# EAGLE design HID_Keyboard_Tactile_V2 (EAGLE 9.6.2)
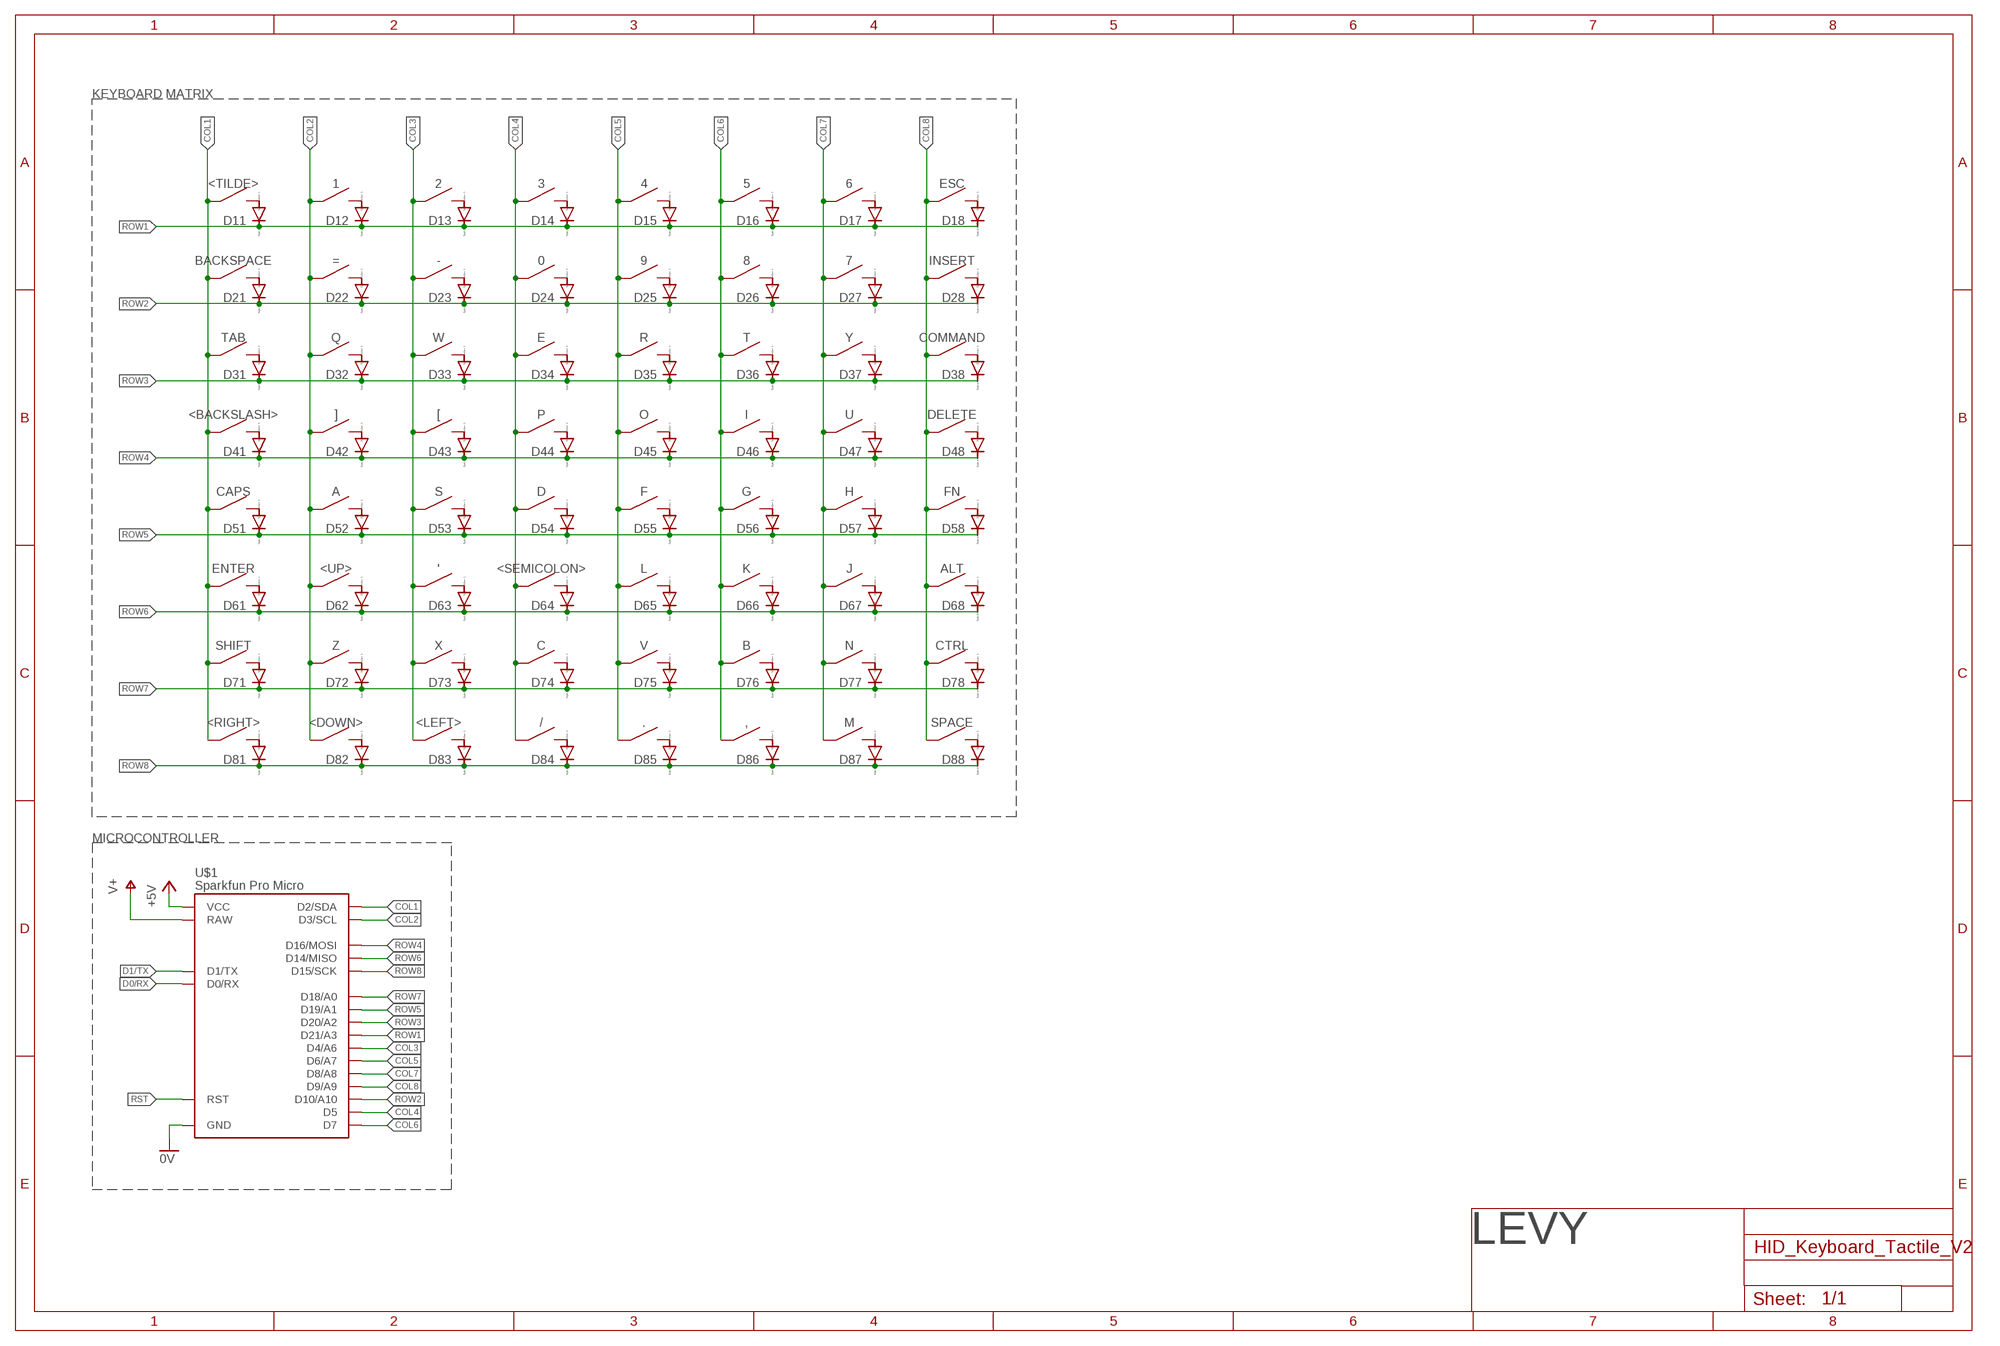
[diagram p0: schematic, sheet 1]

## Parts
0  KEYBOARD_KEYTACTILE_16MM  [KEYBOARD_KEY_TACTILE]
1  KEYBOARD_KEYTACTILE_16MM  [KEYBOARD_KEY_TACTILE]
2  KEYBOARD_KEYTACTILE_16MM  [KEYBOARD_KEY_TACTILE]
3  KEYBOARD_KEYTACTILE_16MM  [KEYBOARD_KEY_TACTILE]
4  KEYBOARD_KEYTACTILE_16MM  [KEYBOARD_KEY_TACTILE]
5  KEYBOARD_KEYTACTILE_16MM  [KEYBOARD_KEY_TACTILE]
6  KEYBOARD_KEYTACTILE_16MM  [KEYBOARD_KEY_TACTILE]
7  KEYBOARD_KEYTACTILE_16MM  [KEYBOARD_KEY_TACTILE]
8  KEYBOARD_KEYTACTILE_16MM  [KEYBOARD_KEY_TACTILE]
9  KEYBOARD_KEYTACTILE_16MM  [KEYBOARD_KEY_TACTILE]
'  KEYBOARD_KEYTACTILE_16MM  [KEYBOARD_KEY_TACTILE]
,  KEYBOARD_KEYTACTILE_16MM  [KEYBOARD_KEY_TACTILE]
-  KEYBOARD_KEYTACTILE_16MM  [KEYBOARD_KEY_TACTILE]
.  KEYBOARD_KEYTACTILE_16MM  [KEYBOARD_KEY_TACTILE]
/  KEYBOARD_KEYTACTILE_16MM  [KEYBOARD_KEY_TACTILE]
<BACKSLASH>  KEYBOARD_KEYTACTILE_16MM  [KEYBOARD_KEY_TACTILE]
<DOWN>  KEYBOARD_KEYTACTILE_16MM  [KEYBOARD_KEY_TACTILE]
<LEFT>  KEYBOARD_KEYTACTILE_16MM  [KEYBOARD_KEY_TACTILE]
<RIGHT>  KEYBOARD_KEYTACTILE_16MM  [KEYBOARD_KEY_TACTILE]
<SEMICOLON>  KEYBOARD_KEYTACTILE_16MM  [KEYBOARD_KEY_TACTILE]
<TILDE>  KEYBOARD_KEYTACTILE_16MM  [KEYBOARD_KEY_TACTILE]
<UP>  KEYBOARD_KEYTACTILE_16MM  [KEYBOARD_KEY_TACTILE]
=  KEYBOARD_KEYTACTILE_16MM  [KEYBOARD_KEY_TACTILE]
[  KEYBOARD_KEYTACTILE_16MM  [KEYBOARD_KEY_TACTILE]
]  KEYBOARD_KEYTACTILE_16MM  [KEYBOARD_KEY_TACTILE]
A  KEYBOARD_KEYTACTILE_16MM  [KEYBOARD_KEY_TACTILE]
ALT  KEYBOARD_KEYTACTILE_16MM  [KEYBOARD_KEY_TACTILE]
B  KEYBOARD_KEYTACTILE_16MM  [KEYBOARD_KEY_TACTILE]
BACKSPACE  KEYBOARD_KEYTACTILE_16MM  [KEYBOARD_KEY_TACTILE]
C  KEYBOARD_KEYTACTILE_16MM  [KEYBOARD_KEY_TACTILE]
CAPS  KEYBOARD_KEYTACTILE_16MM  [KEYBOARD_KEY_TACTILE]
COMMAND  KEYBOARD_KEYTACTILE_16MM  [KEYBOARD_KEY_TACTILE]
CTRL  KEYBOARD_KEYTACTILE_16MM  [KEYBOARD_KEY_TACTILE]
D  KEYBOARD_KEYTACTILE_16MM  [KEYBOARD_KEY_TACTILE]
D11  DIODE-SOD323-W  [SOD323-W]
D12  DIODE-SOD323-W  [SOD323-W]
D13  DIODE-SOD323-W  [SOD323-W]
D14  DIODE-SOD323-W  [SOD323-W]
D15  DIODE-SOD323-W  [SOD323-W]
D16  DIODE-SOD323-W  [SOD323-W]
D17  DIODE-SOD323-W  [SOD323-W]
D18  DIODE-SOD323-W  [SOD323-W]
D21  DIODE-SOD323-W  [SOD323-W]
D22  DIODE-SOD323-W  [SOD323-W]
D23  DIODE-SOD323-W  [SOD323-W]
D24  DIODE-SOD323-W  [SOD323-W]
D25  DIODE-SOD323-W  [SOD323-W]
D26  DIODE-SOD323-W  [SOD323-W]
D27  DIODE-SOD323-W  [SOD323-W]
D28  DIODE-SOD323-W  [SOD323-W]
D31  DIODE-SOD323-W  [SOD323-W]
D32  DIODE-SOD323-W  [SOD323-W]
D33  DIODE-SOD323-W  [SOD323-W]
D34  DIODE-SOD323-W  [SOD323-W]
D35  DIODE-SOD323-W  [SOD323-W]
D36  DIODE-SOD323-W  [SOD323-W]
D37  DIODE-SOD323-W  [SOD323-W]
D38  DIODE-SOD323-W  [SOD323-W]
D41  DIODE-SOD323-W  [SOD323-W]
D42  DIODE-SOD323-W  [SOD323-W]
D43  DIODE-SOD323-W  [SOD323-W]
D44  DIODE-SOD323-W  [SOD323-W]
D45  DIODE-SOD323-W  [SOD323-W]
D46  DIODE-SOD323-W  [SOD323-W]
D47  DIODE-SOD323-W  [SOD323-W]
D48  DIODE-SOD323-W  [SOD323-W]
D51  DIODE-SOD323-W  [SOD323-W]
D52  DIODE-SOD323-W  [SOD323-W]
D53  DIODE-SOD323-W  [SOD323-W]
D54  DIODE-SOD323-W  [SOD323-W]
D55  DIODE-SOD323-W  [SOD323-W]
D56  DIODE-SOD323-W  [SOD323-W]
D57  DIODE-SOD323-W  [SOD323-W]
D58  DIODE-SOD323-W  [SOD323-W]
D61  DIODE-SOD323-W  [SOD323-W]
D62  DIODE-SOD323-W  [SOD323-W]
D63  DIODE-SOD323-W  [SOD323-W]
D64  DIODE-SOD323-W  [SOD323-W]
D65  DIODE-SOD323-W  [SOD323-W]
D66  DIODE-SOD323-W  [SOD323-W]
D67  DIODE-SOD323-W  [SOD323-W]
D68  DIODE-SOD323-W  [SOD323-W]
D71  DIODE-SOD323-W  [SOD323-W]
D72  DIODE-SOD323-W  [SOD323-W]
D73  DIODE-SOD323-W  [SOD323-W]
D74  DIODE-SOD323-W  [SOD323-W]
D75  DIODE-SOD323-W  [SOD323-W]
D76  DIODE-SOD323-W  [SOD323-W]
D77  DIODE-SOD323-W  [SOD323-W]
D78  DIODE-SOD323-W  [SOD323-W]
D81  DIODE-SOD323-W  [SOD323-W]
D82  DIODE-SOD323-W  [SOD323-W]
D83  DIODE-SOD323-W  [SOD323-W]
D84  DIODE-SOD323-W  [SOD323-W]
D85  DIODE-SOD323-W  [SOD323-W]
D86  DIODE-SOD323-W  [SOD323-W]
D87  DIODE-SOD323-W  [SOD323-W]
D88  DIODE-SOD323-W  [SOD323-W]
DELETE  KEYBOARD_KEYTACTILE_16MM  [KEYBOARD_KEY_TACTILE]
E  KEYBOARD_KEYTACTILE_16MM  [KEYBOARD_KEY_TACTILE]
ENTER  KEYBOARD_KEYTACTILE_16MM  [KEYBOARD_KEY_TACTILE]
ESC  KEYBOARD_KEYTACTILE_16MM  [KEYBOARD_KEY_TACTILE]
F  KEYBOARD_KEYTACTILE_16MM  [KEYBOARD_KEY_TACTILE]
FN  KEYBOARD_KEYTACTILE_16MM  [KEYBOARD_KEY_TACTILE]
G  KEYBOARD_KEYTACTILE_16MM  [KEYBOARD_KEY_TACTILE]
H  KEYBOARD_KEYTACTILE_16MM  [KEYBOARD_KEY_TACTILE]
I  KEYBOARD_KEYTACTILE_16MM  [KEYBOARD_KEY_TACTILE]
INSERT  KEYBOARD_KEYTACTILE_16MM  [KEYBOARD_KEY_TACTILE]
J  KEYBOARD_KEYTACTILE_16MM  [KEYBOARD_KEY_TACTILE]
K  KEYBOARD_KEYTACTILE_16MM  [KEYBOARD_KEY_TACTILE]
L  KEYBOARD_KEYTACTILE_16MM  [KEYBOARD_KEY_TACTILE]
M  KEYBOARD_KEYTACTILE_16MM  [KEYBOARD_KEY_TACTILE]
N  KEYBOARD_KEYTACTILE_16MM  [KEYBOARD_KEY_TACTILE]
O  KEYBOARD_KEYTACTILE_16MM  [KEYBOARD_KEY_TACTILE]
P  KEYBOARD_KEYTACTILE_16MM  [KEYBOARD_KEY_TACTILE]
Q  KEYBOARD_KEYTACTILE_16MM  [KEYBOARD_KEY_TACTILE]
R  KEYBOARD_KEYTACTILE_16MM  [KEYBOARD_KEY_TACTILE]
S  KEYBOARD_KEYTACTILE_16MM  [KEYBOARD_KEY_TACTILE]
SHIFT  KEYBOARD_KEYTACTILE_16MM  [KEYBOARD_KEY_TACTILE]
SPACE  KEYBOARD_KEYTACTILE_16MM  [KEYBOARD_KEY_TACTILE]
T  KEYBOARD_KEYTACTILE_16MM  [KEYBOARD_KEY_TACTILE]
TAB  KEYBOARD_KEYTACTILE_16MM  [KEYBOARD_KEY_TACTILE]
U  KEYBOARD_KEYTACTILE_16MM  [KEYBOARD_KEY_TACTILE]
U$1  PROMICRO90PINHEAD  [PROMICRO_90PINHEAD]
U$2  LEVY_LOGOSML  [LEVY_LOGO_NEW_SML]
V  KEYBOARD_KEYTACTILE_16MM  [KEYBOARD_KEY_TACTILE]
W  KEYBOARD_KEYTACTILE_16MM  [KEYBOARD_KEY_TACTILE]
X  KEYBOARD_KEYTACTILE_16MM  [KEYBOARD_KEY_TACTILE]
Y  KEYBOARD_KEYTACTILE_16MM  [KEYBOARD_KEY_TACTILE]
Z  KEYBOARD_KEYTACTILE_16MM  [KEYBOARD_KEY_TACTILE]

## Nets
0V: U$1.GND0(GND) U$1.GND1(GND) U$1.GND3(GND)
+5V: U$1.VCC
COL1: <BACKSLASH>.B <BACKSLASH>.D <RIGHT>.B <RIGHT>.D <TILDE>.B <TILDE>.D BACKSPACE.B BACKSPACE.D CAPS.B CAPS.D ENTER.B ENTER.D SHIFT.B SHIFT.D TAB.B TAB.D U$1.2(D2/SDA)
COL2: 1.B 1.D <DOWN>.B <DOWN>.D <UP>.B <UP>.D =.B =.D ].B ].D A.B A.D Q.B Q.D U$1.3(D3/SCL) Z.B Z.D
COL3: 2.B 2.D '.B '.D -.B -.D <LEFT>.B <LEFT>.D [.B [.D S.B S.D U$1.4(D4/A6) W.B W.D X.B X.D
COL4: 0.B 0.D 3.B 3.D /.B /.D <SEMICOLON>.B <SEMICOLON>.D C.B C.D D.B D.D E.B E.D P.B P.D U$1.5(D5)
COL5: 4.B 4.D 9.B 9.D ..B ..D F.B F.D L.B L.D O.B O.D R.B R.D U$1.6(D6/A7) V.B V.D
COL6: 5.B 5.D 8.B 8.D ,.B ,.D B.B B.D G.B G.D I.B I.D K.B K.D T.B T.D U$1.7(D7)
COL7: 6.B 6.D 7.B 7.D H.B H.D J.B J.D M.B M.D N.B N.D U$1.8(D8/A8) U.B U.D Y.B Y.D
COL8: ALT.B ALT.D COMMAND.B COMMAND.D CTRL.B CTRL.D DELETE.B DELETE.D ESC.B ESC.D FN.B FN.D INSERT.B INSERT.D SPACE.B SPACE.D U$1.9(D9/A9)
D0/RX: U$1.0(D0/RX)
D1/TX: U$1.1(D1/TX)
N$1: <TILDE>.A <TILDE>.C D11.A
N$2: 1.A 1.C D12.A
N$3: 2.A 2.C D13.A
N$4: 3.A 3.C D14.A
N$5: 4.A 4.C D15.A
N$6: 5.A 5.C D16.A
N$7: 6.A 6.C D17.A
N$8: 7.A 7.C D27.A
N$9: 8.A 8.C D26.A
N$10: 9.A 9.C D25.A
N$11: 0.A 0.C D24.A
N$12: -.A -.C D23.A
N$13: =.A =.C D22.A
N$14: BACKSPACE.A BACKSPACE.C D21.A
N$15: D31.A TAB.A TAB.C
N$16: D32.A Q.A Q.C
N$17: D33.A W.A W.C
N$18: D34.A E.A E.C
N$19: D35.A R.A R.C
N$20: D36.A T.A T.C
N$21: D37.A Y.A Y.C
N$22: D47.A U.A U.C
N$23: D46.A I.A I.C
N$24: D45.A O.A O.C
N$25: D44.A P.A P.C
N$26: [.A [.C D43.A
N$27: ].A ].C D42.A
N$28: <BACKSLASH>.A <BACKSLASH>.C D41.A
N$29: CAPS.A CAPS.C D51.A
N$30: A.A A.C D52.A
N$31: D53.A S.A S.C
N$32: D54.A D.A D.C
N$33: D55.A F.A F.C
N$34: D56.A G.A G.C
N$35: D57.A H.A H.C
N$36: D67.A J.A J.C
N$37: D66.A K.A K.C
N$38: D65.A L.A L.C
N$39: <SEMICOLON>.A <SEMICOLON>.C D64.A
N$40: '.A '.C D63.A
N$41: D61.A ENTER.A ENTER.C
N$42: D71.A SHIFT.A SHIFT.C
N$43: D88.A SPACE.A SPACE.C
N$44: D72.A Z.A Z.C
N$45: CTRL.A CTRL.C D78.A
N$46: D73.A X.A X.C
N$47: ALT.A ALT.C D68.A
N$48: C.A C.C D74.A
N$49: D58.A FN.A FN.C
N$50: D75.A V.A V.C
N$51: D48.A DELETE.A DELETE.C
N$52: B.A B.C D76.A
N$53: D77.A N.A N.C
N$54: D87.A M.A M.C
N$55: ,.A ,.C D86.A
N$56: D18.A ESC.A ESC.C
N$57: ..A ..C D85.A
N$58: D28.A INSERT.A INSERT.C
N$59: /.A /.C D84.A
N$60: COMMAND.A COMMAND.C D38.A
N$61: <LEFT>.A <LEFT>.C D83.A
N$62: <UP>.A <UP>.C D62.A
N$63: <DOWN>.A <DOWN>.C D82.A
N$64: <RIGHT>.A <RIGHT>.C D81.A
ROW1: D11.C D12.C D13.C D14.C D15.C D16.C D17.C D18.C U$1.21(D21/A3)
ROW2: D21.C D22.C D23.C D24.C D25.C D26.C D27.C D28.C U$1.10(D10/A10)
ROW3: D31.C D32.C D33.C D34.C D35.C D36.C D37.C D38.C U$1.20(D20/A2)
ROW4: D41.C D42.C D43.C D44.C D45.C D46.C D47.C D48.C U$1.16(D16/MOSI)
ROW5: D51.C D52.C D53.C D54.C D55.C D56.C D57.C D58.C U$1.19(D19/A1)
ROW6: D61.C D62.C D63.C D64.C D65.C D66.C D67.C D68.C U$1.14(D14/MISO)
ROW7: D71.C D72.C D73.C D74.C D75.C D76.C D77.C D78.C U$1.18(D18/A0)
ROW8: D81.C D82.C D83.C D84.C D85.C D86.C D87.C D88.C U$1.15(D15/SCK)
RST: U$1.RST
V+: U$1.RAW

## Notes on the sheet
- KEYBOARD MATRIX
- MICROCONTROLLER

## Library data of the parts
0 1-9 ' , - . / <BACKSLASH> <DOWN> <LEFT> <RIGHT> <SEMICOLON> <TILDE> <UP> = [ ] A ALT B BACKSPACE C CAPS COMMAND CTRL D DELETE E ENTER ESC F FN G H I INSERT J K L M N O P Q R S SHIFT SPACE T TAB U V W X Y Z = LEVY_COMPONENTS:KEYBOARD_KEY
D11-D18 D21-D28 D31-D38 D41-D48 D51-D58 D61-D68 D71-D78 D81-D88 = diode:DIODE-: DIODE
U$1 = LEVY_DevBoards:PROMICRO
U$2 = LEVY_COMPONENTS:LEVY_LOGO

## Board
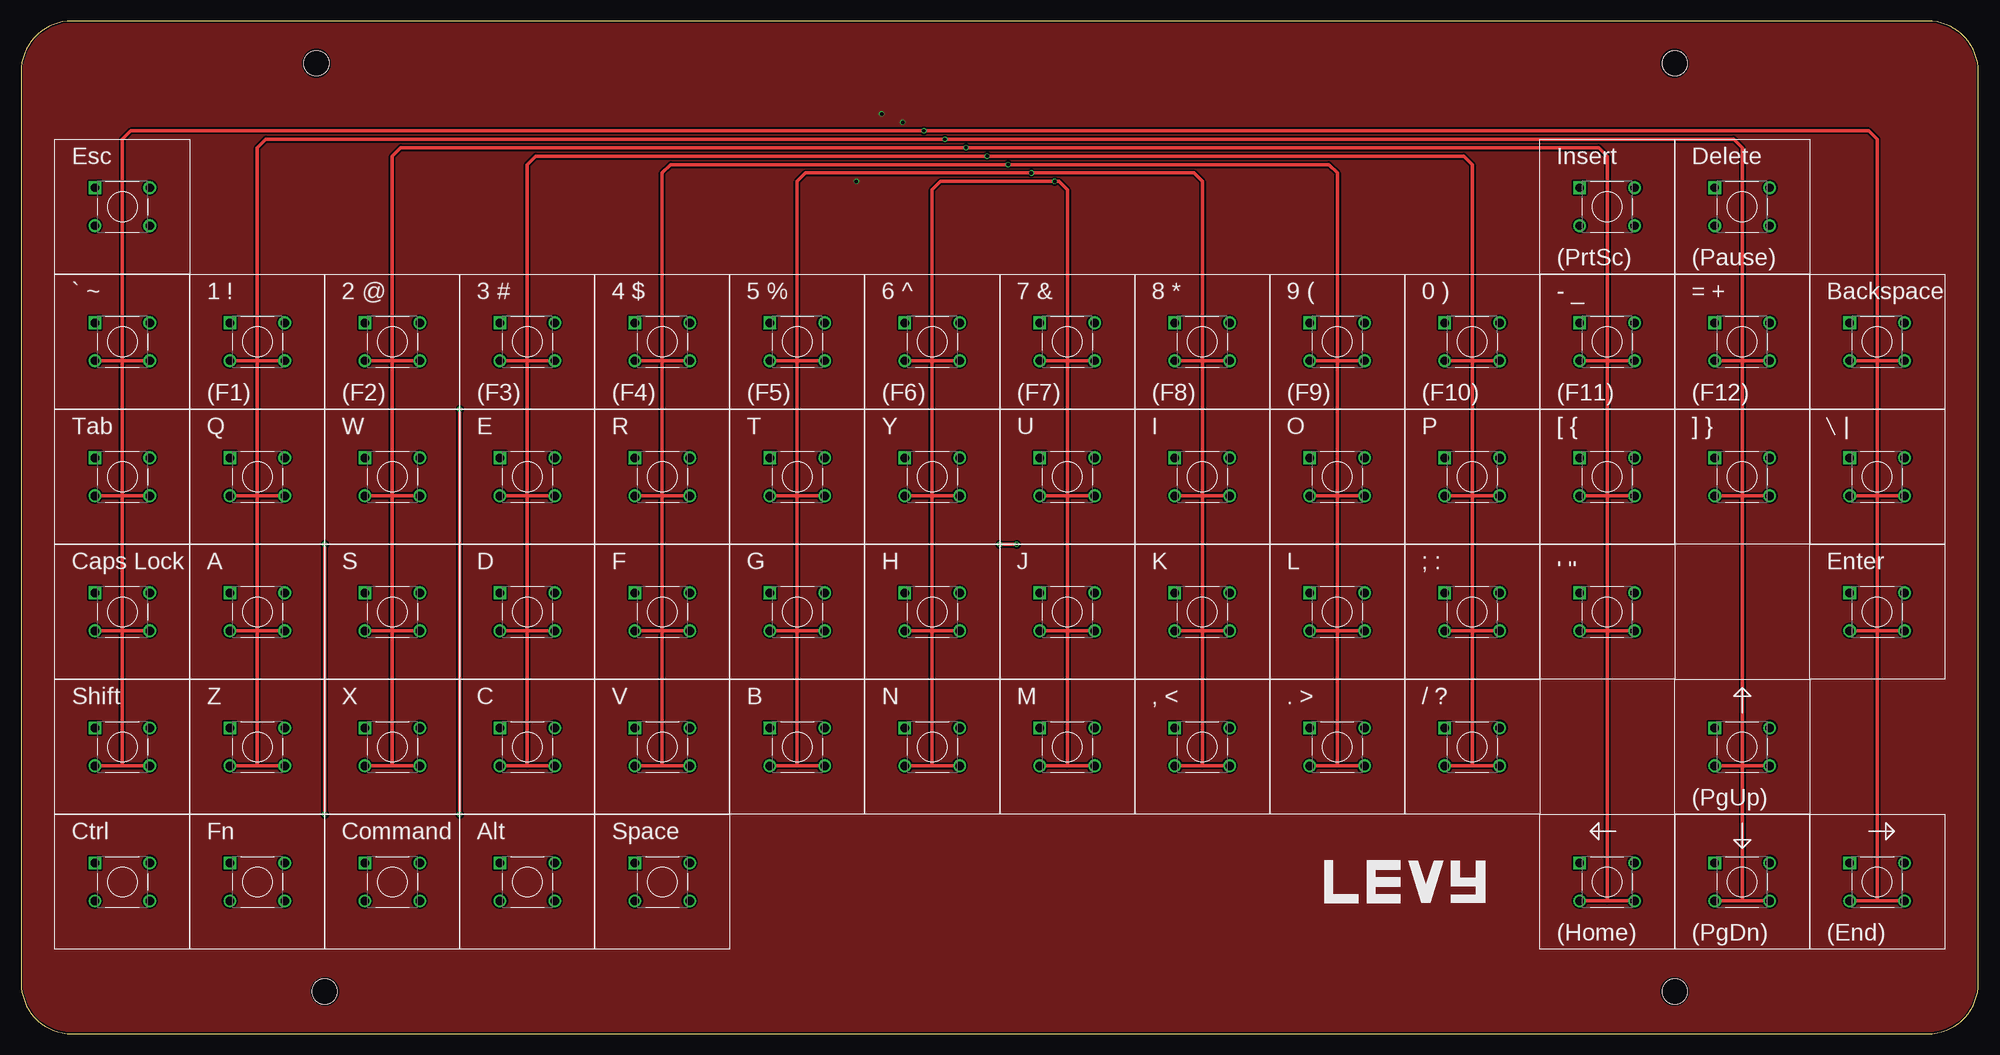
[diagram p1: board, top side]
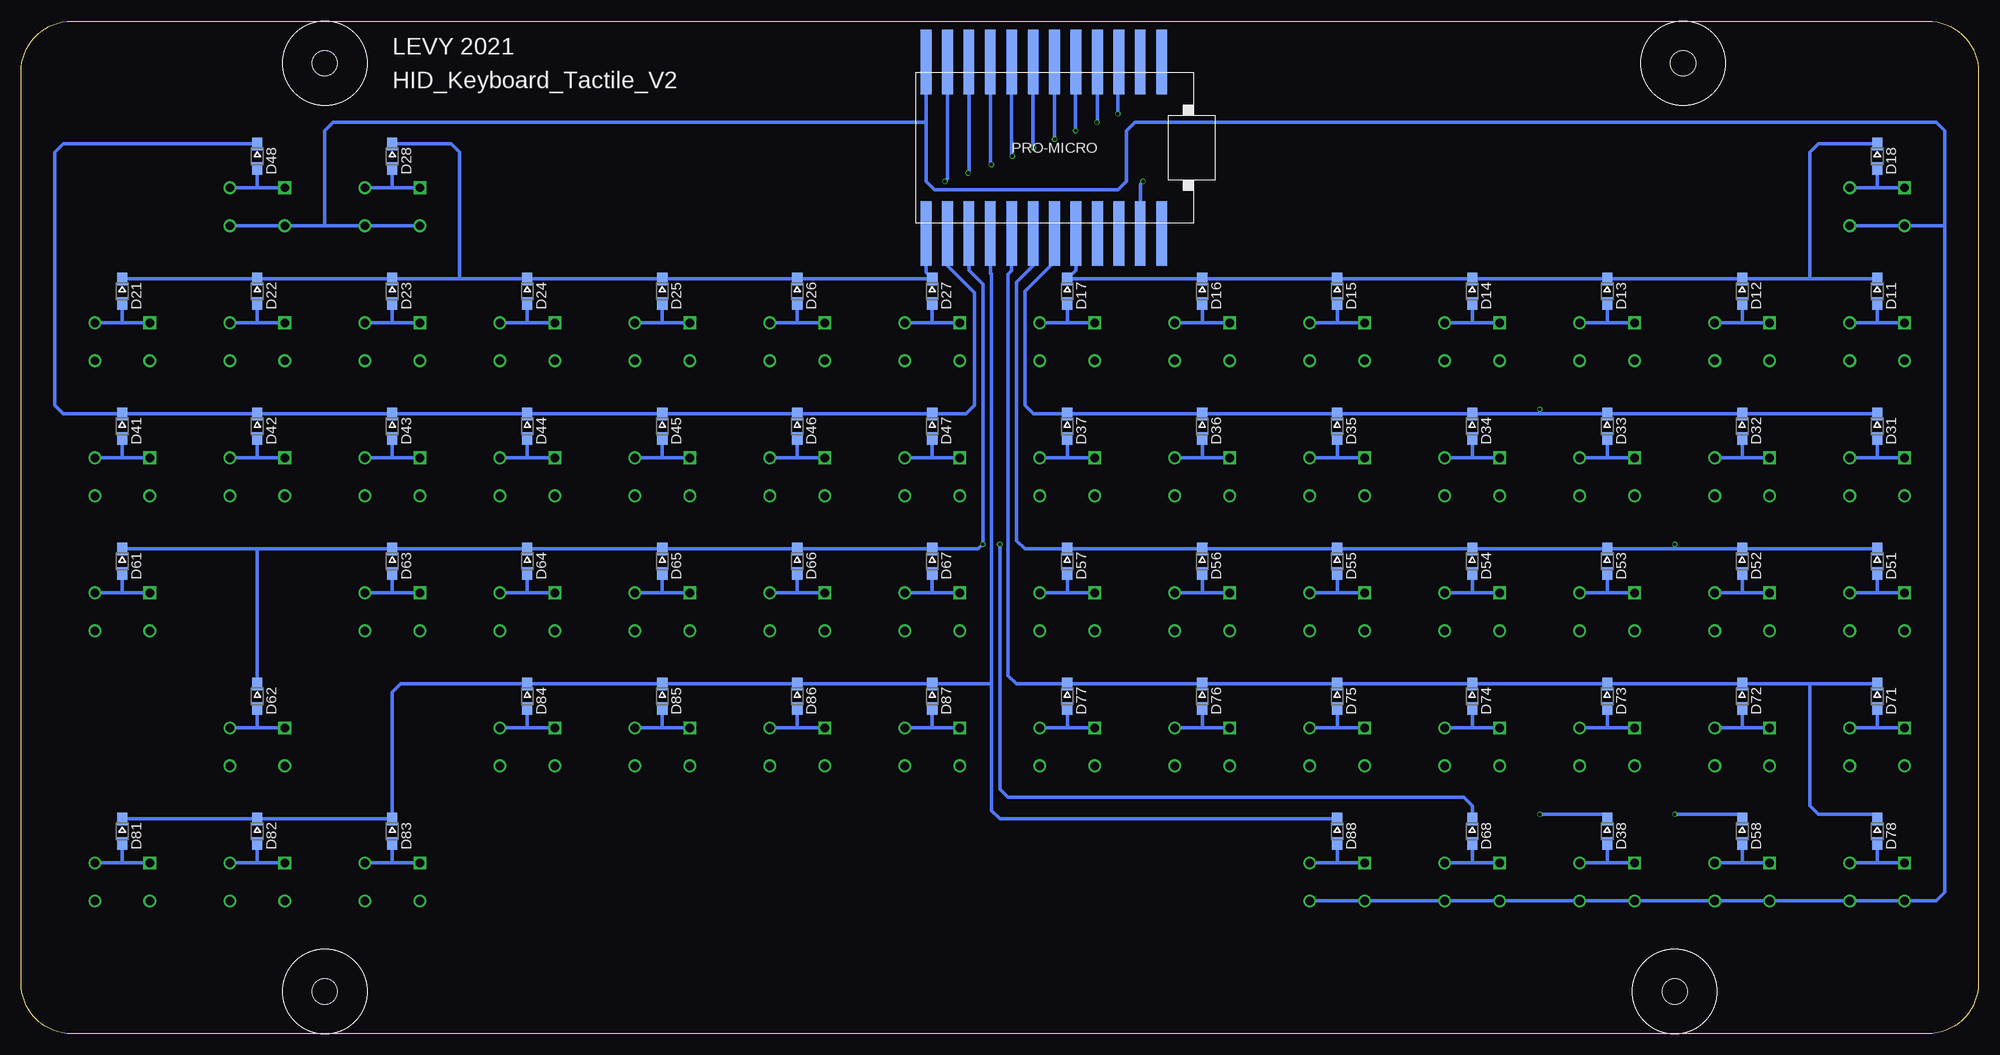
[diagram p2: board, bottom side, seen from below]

Size 232 x 120 mm. Coordinates in mm from the lower left corner, seen from the top.
Outline: 226,120 6,120 arc90 0,114 0,6 arc90 6,0 226,0 arc90 232,6 232,114 arc90 226,120
Copper layers (1*16): Top 0.035559375mm / dielectric 1.6mm / Bottom 0.035559375mm
Design rules "JLCPCB_1.6mm_2Layer": minimum track width 5mil, minimum drill 12mil, track to track 5mil, track to pad 5mil, pad to pad 5mil, via to via 5mil, smd to smd 5mil, copper to edge 8mil, drill to drill 6mil, minimum pad ring 5mil, minimum via ring 3mil, stop-mask expansion 2.5mil, vias tented up to drill 0mil, thermal gap 10mil
Holes 3 mm at 36,5 196,5 35,115 196,115

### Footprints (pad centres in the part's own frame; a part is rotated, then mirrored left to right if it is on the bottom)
KEYBOARD_KEY_TACTILE = drill 1 square: A -3.25,2.25 | drill 1: B -3.25,-2.25; C 3.25,2.25; D 3.25,-2.25
SOD323-W = smd 1.5 x 1.2: A 1.45,0; C -1.45,0
PROMICRO_90PINHEAD = smd 1.27 x 7.62: 0 -10.16,-10.16; 1 -12.7,-10.16; 2 -2.54,-10.16; 3 0,-10.16; 4 2.54,-10.16; 5 5.08,-10.16; 6 7.62,-10.16; 7 10.16,-10.16; 8 12.7,-10.16; 9 15.24,-10.16; 10 15.24,10.16; 14 10.16,10.16; 15 7.62,10.16; 16 12.7,10.16; 18 5.08,10.16; 19 2.54,10.16; 20 0,10.16; 21 -2.54,10.16; GND0 -7.62,-10.16; GND1 -5.08,-10.16; GND3 -10.16,10.16; RAW -12.7,10.16; RST -7.62,10.16; VCC -5.08,10.16

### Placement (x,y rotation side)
0  172,82 0 top
1  28,82 0 top
2  44,82 0 top
3  60,82 0 top
4  76,82 0 top
5  92,82 0 top
6  108,82 0 top
7  124,82 0 top
8  140,82 0 top
9  156,82 0 top
'  188,50 0 top
,  140,34 0 top
-  188,82 0 top
.  156,34 0 top
/  172,34 0 top
<BACKSLASH>  220,66 0 top
<DOWN>  204,18 0 top
<LEFT>  188,18 0 top
<RIGHT>  220,18 0 top
<SEMICOLON>  172,50 0 top
<TILDE>  12,82 0 top
<UP>  204,34 0 top
=  204,82 0 top
[  188,66 0 top
]  204,66 0 top
A  28,50 0 top
ALT  60,18 0 top
B  92,34 0 top
BACKSPACE  220,82 0 top
C  60,34 0 top
CAPS  12,50 0 top
COMMAND  44,18 0 top
CTRL  12,18 0 top
D  60,50 0 top
D11  12,88 270 bottom
D12  28,88 270 bottom
D13  44,88 270 bottom
D14  60,88 270 bottom
D15  76,88 270 bottom
D16  92,88 270 bottom
D17  108,88 270 bottom
D18  12,104 270 bottom
D21  220,88 270 bottom
D22  204,88 270 bottom
D23  188,88 270 bottom
D24  172,88 270 bottom
D25  156,88 270 bottom
D26  140,88 270 bottom
D27  124,88 270 bottom
D28  188,104 270 bottom
D31  12,72 270 bottom
D32  28,72 270 bottom
D33  44,72 270 bottom
D34  60,72 270 bottom
D35  76,72 270 bottom
D36  92,72 270 bottom
D37  108,72 270 bottom
D38  44,24 270 bottom
D41  220,72 270 bottom
D42  204,72 270 bottom
D43  188,72 270 bottom
D44  172,72 270 bottom
D45  156,72 270 bottom
D46  140,72 270 bottom
D47  124,72 270 bottom
D48  204,104 270 bottom
D51  12,56 270 bottom
D52  28,56 270 bottom
D53  44,56 270 bottom
D54  60,56 270 bottom
D55  76,56 270 bottom
D56  92,56 270 bottom
D57  108,56 270 bottom
D58  28,24 270 bottom
D61  220,56 270 bottom
D62  204,40 270 bottom
D63  188,56 270 bottom
D64  172,56 270 bottom
D65  156,56 270 bottom
D66  140,56 270 bottom
D67  124,56 270 bottom
D68  60,24 270 bottom
D71  12,40 270 bottom
D72  28,40 270 bottom
D73  44,40 270 bottom
D74  60,40 270 bottom
D75  76,40 270 bottom
D76  92,40 270 bottom
D77  108,40 270 bottom
D78  12,24 270 bottom
D81  220,24 270 bottom
D82  204,24 270 bottom
D83  188,24 270 bottom
D84  172,40 270 bottom
D85  156,40 270 bottom
D86  140,40 270 bottom
D87  124,40 270 bottom
D88  76,24 270 bottom
DELETE  204,98 0 top
E  60,66 0 top
ENTER  220,50 0 top
ESC  12,98 0 top
F  76,50 0 top
FN  28,18 0 top
G  92,50 0 top
H  108,50 0 top
I  140,66 0 top
INSERT  188,98 0 top
J  124,50 0 top
K  140,50 0 top
L  156,50 0 top
M  124,34 0 top
N  108,34 0 top
O  156,66 0 top
P  172,66 0 top
Q  28,66 0 top
R  76,66 0 top
S  44,50 0 top
SHIFT  12,34 0 top
SPACE  76,18 0 top
T  92,66 0 top
TAB  12,66 0 top
U  124,66 0 top
U$1  109.5,105 180 bottom
U$2  164,18.5 0 top
V  76,34 0 top
W  44,66 0 top
X  44,34 0 top
Y  108,66 0 top
Z  28,34 0 top

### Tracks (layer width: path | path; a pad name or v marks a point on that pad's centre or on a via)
0V  (via drill 0.4)
  Bottom 0.406: U$1.GND3 99.34,100.66 v99,101 | U$1.GND0 102,115.04 v102,109 | U$1.GND1 104.42,108.08 v104.5,108
  pour Top (isolate 0.2): 0,120 232,120 232,0 0,0
COL1  (via drill 0.4)
  Top 0.406: <TILDE>.B 12,79.75 | 12,79.75 <TILDE>.D | TAB.B 12,63.75 | TAB.D 12,63.75 | CAPS.B 12,47.75 | CAPS.D 12,47.75 | SHIFT.B 12,31.75 | 12,31.75 SHIFT.D | BACKSPACE.B 220,79.75 | BACKSPACE.D 220,79.75 | <BACKSLASH>.D 220,63.75 | <BACKSLASH>.B 220,63.75 | ENTER.B 220,47.75 | ENTER.D 220,47.75 | <RIGHT>.B 220,15.75 | 220,15.75 <RIGHT>.D | 220,15.75 220,47.75 | 220,47.75 220,63.75 | 220,63.75 220,79.75 | 12,31.75 12,47.75 | 12,47.75 12,63.75 | 12,63.75 12,79.75 | 220,79.75 220,106 219,107 v107,107 13,107 12,106 12,79.75
  Bottom 0.406: U$1.2 107,115.12 v107,107
COL2  (via drill 0.4)
  Top 0.406: Z.B 28,31.75 | 28,31.75 Z.D | A.B 28,47.75 | A.D 28,47.75 | Q.B 28,63.75 | 28,63.75 Q.D | 1.B 28,79.75 | 28,79.75 1.D | =.D 204,79.75 | 204,79.75 =.B | ].B 204,63.75 | 204,63.75 ].D | <UP>.D 204,31.75 | 204,31.75 <UP>.B | <DOWN>.B 204,15.75 | 204,15.75 <DOWN>.D | 204,79.75 204,63.75 | 204,63.75 204,31.75 | 204,31.75 204,15.75 | 28,31.75 28,47.75 | 28,47.75 28,63.75 | 28,63.75 28,79.75 | 28,79.75 28,105 29,106 v109.5,106 203,106 204,105 204,79.75
  Bottom 0.406: U$1.3 v109.5,106
COL3  (via drill 0.4)
  Top 0.406: 2.B 44,79.75 | 2.D 44,79.75 | W.D 44,63.75 | W.B 44,63.75 | S.B 44,47.75 | 44,47.75 S.D | X.D 44,31.75 | 44,31.75 X.B | -.B 188,79.75 | 188,79.75 -.D | [.D 188,63.75 | [.B 188,63.75 | '.B 188,47.75 | 188,47.75 '.D | <LEFT>.D 188,15.75 | 188,15.75 <LEFT>.B | 188,15.75 188,47.75 | 188,47.75 188,63.75 | 188,63.75 188,79.75 | 44,31.75 44,47.75 | 44,47.75 44,63.75 | 44,63.75 44,79.75 | 44,79.75 44,104 45,105 v112,105 187,105 188,104 188,79.75
  Bottom 0.406: U$1.4 112.04,105 v112,105
COL4  (via drill 0.4)
  Top 0.406: 3.B 60,79.75 | 60,79.75 3.D | E.D 60,63.75 | 60,63.75 E.B | D.B 60,47.75 | 60,47.75 D.D | C.D 60,31.75 | 60,31.75 C.B | /.D 172,31.75 | 172,31.75 /.B | <SEMICOLON>.B 172,47.75 | <SEMICOLON>.D 172,47.75 | P.D 172,63.75 | P.B 172,63.75 | 0.B 172,79.75 | 172,79.75 0.D | 172,79.75 172,63.75 | 172,63.75 172,47.75 | 172,47.75 172,31.75 | 60,31.75 60,47.75 | 60,47.75 60,63.75 | 60,63.75 60,79.75 | 60,79.75 60,103 61,104 v114.5,104 171,104 172,103 172,79.75
  Bottom 0.406: U$1.5 114.58,104 v114.5,104
COL5  (via drill 0.4)
  Top 0.406: V.B 76,31.75 | 76,31.75 V.D | F.D 76,47.75 | 76,47.75 F.B | R.B 76,63.75 | 76,63.75 R.D | 4.D 76,79.75 | 4.B 76,79.75 | 9.B 156,79.75 | 156,79.75 9.D | O.D 156,63.75 | O.B 156,63.75 | L.B 156,47.75 | L.D 156,47.75 | ..D 156,31.75 | 156,31.75 ..B | 156,31.75 156,47.75 | 156,47.75 156,63.75 | 156,63.75 156,79.75 | 76,31.75 76,47.75 | 76,47.75 76,63.75 | 76,63.75 76,79.75 | 76,79.75 76,102 77,103 v117,103 155,103 156,102 156,79.75
  Bottom 0.406: U$1.6 117.12,103 v117,103
COL6  (via drill 0.4)
  Top 0.406: 5.B 92,79.75 | 5.D 92,79.75 | T.D 92,63.75 | T.B 92,63.75 | G.B 92,47.75 | G.D 92,47.75 | B.D 92,31.75 | 92,31.75 B.B | 8.B 140,79.75 | 140,79.75 8.D | I.D 140,63.75 | I.B 140,63.75 | K.B 140,47.75 | 140,47.75 K.D | ,.D 140,31.75 | 140,31.75 ,.B | 140,79.75 140,63.75 | 140,63.75 140,47.75 | 140,47.75 140,31.75 | 92,31.75 92,47.75 | 92,47.75 92,63.75 | 92,63.75 92,79.75 | 92,79.75 92,101 93,102 v119.75,102 139,102 140,101 140,79.75
  Bottom 0.406: U$1.7 119.66,102 v119.75,102
COL7  (via drill 0.4)
  Top 0.406: N.B 108,31.75 | 108,31.75 N.D | H.D 108,47.75 | H.B 108,47.75 | Y.B 108,63.75 | Y.D 108,63.75 | 6.B 108,79.75 | 6.D 108,79.75 | 7.B 124,79.75 | 124,79.75 7.D | U.D 124,63.75 | U.B 124,63.75 | J.B 124,47.75 | J.D 124,47.75 | M.D 124,31.75 | 124,31.75 M.B | 124,31.75 124,47.75 | 124,47.75 124,63.75 | 124,63.75 124,79.75 | 108,31.75 108,47.75 | 108,47.75 108,63.75 | 108,63.75 108,79.75 | 108,79.75 108,100 109,101 v122.5,101 123,101 124,100 124,79.75
  Bottom 0.406: U$1.8 122.2,101.3 v122.5,101
COL8
  Bottom 0.406: SPACE.D SPACE.B ALT.D ALT.B COMMAND.D COMMAND.B FN.D FN.B CTRL.D CTRL.B 5,15.75 4,16.75 4,95.75 | DELETE.D DELETE.B 196,95.75 | ESC.D ESC.B 4,95.75 | 196,95.75 INSERT.D INSERT.B | U$1.9 124.74,108 | 124.74,108 124.74,101 123.74,100 102,100 101,101 101,107 100,108 5,108 4,107 4,95.75 | 196,95.75 196,107 195,108 124.74,108
N$1
  Bottom 0.406: <TILDE>.A 12,84.25 | 12,84.25 <TILDE>.C | D11.A 12,84.25
N$2
  Bottom 0.406: 1.A 28,84.25 | 28,84.25 1.C | D12.A 28,84.25
N$3
  Bottom 0.406: 2.A 44,84.25 | 44,84.25 2.C | D13.A 44,84.25
N$4
  Bottom 0.406: 3.A 60,84.25 | 60,84.25 3.C | D14.A 60,84.25
N$5
  Bottom 0.406: 4.A 76,84.25 | 76,84.25 4.C | D15.A 76,84.25
N$6
  Bottom 0.406: 5.A 92,84.25 | 92,84.25 5.C | D16.A 92,84.25
N$7
  Bottom 0.406: 6.A 108,84.25 | 108,84.25 6.C | D17.A 108,84.25
N$8
  Bottom 0.406: 7.A 124,84.25 | 124,84.25 7.C | D27.A 124,84.25
N$9
  Bottom 0.406: 8.A 140,84.25 | 140,84.25 8.C | D26.A 140,84.25
N$10
  Bottom 0.406: 9.A 156,84.25 | 156,84.25 9.C | D25.A 156,84.25
N$11
  Bottom 0.406: 0.A 172,84.25 | 172,84.25 0.C | D24.A 172,84.25
N$12
  Bottom 0.406: -.A 188,84.25 | 188,84.25 -.C | D23.A 188,84.25
N$13
  Bottom 0.406: =.A 204,84.25 | 204,84.25 =.C | D22.A 204,84.25
N$14
  Bottom 0.406: BACKSPACE.A 220,84.25 | 220,84.25 BACKSPACE.C | D21.A 220,84.25
N$15
  Bottom 0.406: TAB.A 12,68.25 | 12,68.25 TAB.C | D31.A 12,68.25
N$16
  Bottom 0.406: Q.A 28,68.25 | 28,68.25 Q.C | D32.A 28,68.25
N$17
  Bottom 0.406: W.A 44,68.25 | 44,68.25 W.C | D33.A 44,68.25
N$18
  Bottom 0.406: E.A 60,68.25 | 60,68.25 E.C | D34.A 60,68.25
N$19
  Bottom 0.406: R.A 76,68.25 | 76,68.25 R.C | D35.A 76,68.25
N$20
  Bottom 0.406: T.A 92,68.25 | 92,68.25 T.C | D36.A 92,68.25
N$21
  Bottom 0.406: Y.A 108,68.25 | 108,68.25 Y.C | D37.A 108,68.25
N$22
  Bottom 0.406: U.A 124,68.25 | 124,68.25 U.C | D47.A 124,68.25
N$23
  Bottom 0.406: I.A 140,68.25 | 140,68.25 I.C | D46.A 140,68.25
N$24
  Bottom 0.406: O.A 156,68.25 | 156,68.25 O.C | D45.A 156,68.25
N$25
  Bottom 0.406: P.A 172,68.25 | 172,68.25 P.C | D44.A 172,68.25
N$26
  Bottom 0.406: [.A 188,68.25 | 188,68.25 [.C | D43.A 188,68.25
N$27
  Bottom 0.406: ].A 204,68.25 | 204,68.25 ].C | D42.A 204,68.25
N$28
  Bottom 0.406: <BACKSLASH>.A 220,68.25 | 220,68.25 <BACKSLASH>.C | D41.A 220,68.25
N$29
  Bottom 0.406: CAPS.A 12,52.25 | 12,52.25 CAPS.C | D51.A 12,52.25
N$30
  Bottom 0.406: A.A 28,52.25 | 28,52.25 A.C | D52.A 28,52.25
N$31
  Bottom 0.406: S.A 44,52.25 | 44,52.25 S.C | D53.A 44,52.25
N$32
  Bottom 0.406: D.A 60,52.25 | 60,52.25 D.C | D54.A 60,52.25
N$33
  Bottom 0.406: F.A 76,52.25 | 76,52.25 F.C | D55.A 76,52.25
N$34
  Bottom 0.406: G.A 92,52.25 | 92,52.25 G.C | D56.A 92,52.25
N$35
  Bottom 0.406: H.A 108,52.25 | 108,52.25 H.C | D57.A 108,52.25
N$36
  Bottom 0.406: J.A 124,52.25 | 124,52.25 J.C | D67.A 124,52.25
N$37
  Bottom 0.406: K.A 140,52.25 | 140,52.25 K.C | D66.A 140,52.25
N$38
  Bottom 0.406: L.A 156,52.25 | 156,52.25 L.C | D65.A 156,52.25
N$39
  Bottom 0.406: <SEMICOLON>.A 172,52.25 | 172,52.25 <SEMICOLON>.C | D64.A 172,52.25
N$40
  Bottom 0.406: '.A 188,52.25 | 188,52.25 '.C | D63.A 188,52.25
N$41
  Bottom 0.406: ENTER.A 220,52.25 | 220,52.25 ENTER.C | D61.A 220,52.25
N$42
  Bottom 0.406: SHIFT.A 12,36.25 | 12,36.25 SHIFT.C | D71.A 12,36.25
N$43
  Bottom 0.406: SPACE.A 76,20.25 | 76,20.25 SPACE.C | D88.A 76,20.25
N$44
  Bottom 0.406: Z.A 28,36.25 | 28,36.25 Z.C | D72.A 28,36.25
N$45
  Bottom 0.406: CTRL.C 12,20.25 | 12,20.25 CTRL.A | D78.A 12,20.25
N$46
  Bottom 0.406: X.A 44,36.25 | 44,36.25 X.C | D73.A 44,36.25
N$47
  Bottom 0.406: ALT.A 60,20.25 | 60,20.25 ALT.C | D68.A 60,20.25
N$48
  Bottom 0.406: C.A 60,36.25 | 60,36.25 C.C | D74.A 60,36.25
N$49
  Bottom 0.406: FN.A 28,20.25 | 28,20.25 FN.C | D58.A 28,20.25
N$50
  Bottom 0.406: V.A 76,36.25 | 76,36.25 V.C | D75.A 76,36.25
N$51
  Bottom 0.406: DELETE.A 204,100.25 | 204,100.25 DELETE.C | D48.A 204,100.25
N$52
  Bottom 0.406: B.A 92,36.25 | 92,36.25 B.C | D76.A 92,36.25
N$53
  Bottom 0.406: N.A 108,36.25 | 108,36.25 N.C | D77.A 108,36.25
N$54
  Bottom 0.406: M.A 124,36.25 | 124,36.25 M.C | D87.A 124,36.25
N$55
  Bottom 0.406: ,.A 140,36.25 | 140,36.25 ,.C | D86.A 140,36.25
N$56
  Bottom 0.406: ESC.A 12,100.25 | 12,100.25 ESC.C | D18.A 12,100.25
N$57
  Bottom 0.406: ..A 156,36.25 | 156,36.25 ..C | D85.A 156,36.25
N$58
  Bottom 0.406: INSERT.A 188,100.25 | 188,100.25 INSERT.C | D28.A 188,100.25
N$59
  Bottom 0.406: /.A 172,36.25 | 172,36.25 /.C | D84.A 172,36.25
N$60
  Bottom 0.406: COMMAND.A 44,20.25 | 44,20.25 COMMAND.C | D38.A 44,20.25
N$61
  Bottom 0.406: <LEFT>.A 188,20.25 | 188,20.25 <LEFT>.C | D83.A 188,20.25
N$62
  Bottom 0.406: <UP>.A 204,36.25 | 204,36.25 <UP>.C | D62.A 204,36.25
N$63
  Bottom 0.406: <DOWN>.A 204,20.25 | 204,20.25 <DOWN>.C | D82.A 204,20.25
N$64
  Bottom 0.406: <RIGHT>.A 220,20.25 | 220,20.25 <RIGHT>.C | D81.A 220,20.25
ROW1
  Bottom 0.406: D11.C 20,89.45 | 20,89.45 D12.C D13.C D14.C D15.C D16.C D17.C 108,89.5 107.96,89.5 106.96,90.5 U$1.21 | D18.C 19,105.45 20,104.45 20,89.45
ROW2
  Bottom 0.406: D21.C D22.C D23.C 180,89.45 | 180,89.45 D24.C D25.C D26.C D27.C 124,89.5 124.74,90.24 U$1.10 | D28.C 181,105.45 180,104.45 180,89.45
ROW3  (via drill 0.4)
  Top 0.406: v52,26 v52,74
  Bottom 0.406: 52,73.45 D34.C D35.C D36.C D37.C 112,73.45 113,74.45 113,88 109.5,91.5 U$1.20 | 52,73.45 D33.C D32.C D31.C | 52,73.45 v52,74 | D38.C 44,26 v52,26
ROW4
  Bottom 0.406: U$1.16 122.2,91 119,87.8 119,74.45 120,73.45 D47.C D46.C D45.C D44.C D43.C D42.C D41.C 227,73.45 228,74.45 228,104.45 227,105.45 D48.C
ROW5  (via drill 0.4)
  Top 0.406: v36,26 v36,58
  Bottom 0.406: 36,57.45 D53.C D54.C D55.C D56.C D57.C 113,57.45 114,58.45 114,89.04 112.04,91 U$1.19 | 36,57.45 D52.C D51.C | 36,57.45 v36,58 | D58.C 28,26 v36,26
ROW6  (via drill 0.4)
  Top 0.406: v116,58 v118,58
  Bottom 0.406: D61.C 204,57.45 | 204,57.45 D63.C D64.C D65.C D66.C D67.C 118.55,57.45 v118,58 118,88.84 119.66,90.5 U$1.14 | D62.C 204,57.45 | D68.C 60,27 61,28 115,28 116,29 v116,58
ROW7
  Bottom 0.406: 20,41.45 D72.C D73.C D74.C D75.C D76.C D77.C 114,41.45 115,42.45 115,90 114.58,90.42 U$1.18 | 20,41.45 D71.C | D78.C 12,26 19,26 20,27 20,41.45
ROW8
  Bottom 0.406: D81.C D82.C D83.C 188,40.45 187,41.45 D84.C D85.C D86.C D87.C 117,41.45 | U$1.15 117.12,90.09 117,90.09 117,41.45 | D88.C 116,25.45 117,26.45 117,41.45

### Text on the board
tNames: Esc | Insert | Delete | (PrtSc) | (Pause) | ` ~ | 1 ! | 2 @ | 3 # | 4 $ | 5 % | 6 ^ | 7 & | 8 * | 9 ( | 0 ) | - _ | = + | Backspace | (F1) | (F2) | (F3) | (F4) | (F5) | (F6) | (F7) | (F8) | (F9) | (F10) | (F11) | (F12) | Tab | [ { | ] } | | | Caps Lock | ; : | Enter | ' " | Shift | , < | . > | / ? | (PgUp) | Ctrl | Fn | Command | Alt | Space | (Home) | (PgDn) | (End)
bNames: LEVY 2021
